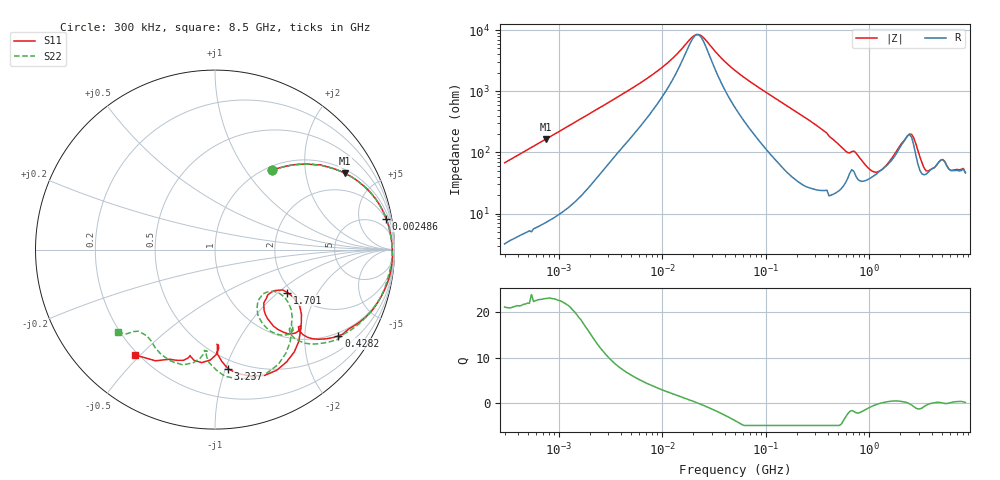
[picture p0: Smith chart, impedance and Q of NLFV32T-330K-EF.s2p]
! S-parameter Generated by TDK Corporation
! Copyright(C) 2015 TDK Corporation.
! All Rights Reserved.
! TDK P/N: NLFV32T-330K-EF (Inductors)
! Property: L=33uH at 2.52MHz
! Size(LxWxT): 3.2x2.5x2.2mm, 0.126x0.098x0.087inches
! Model Type: s2p (Touchstone File Format Version 1.0)
! Frequency: DC=Yes Start=0.3MHz Stop=8500MHz 225points Log-sweep
! Note:
! Model Generated on Jun. 23, 2015
! Hash(MD5):
! Port Assignments:
!  1 ---@@@--- 2
! Applicable Conditions:
!  Temperature = 25 degC
!  DC Bias Current = 0 A
!  Small Signal Operation
! Terms and conditions regarding TDK Simulation Models
! (1)This simulation model is being provided solely for informational purposes. Please refer to the specifications of the products in terms of detailed characteristics of such products.
! (2)In no event shall TDK Corporation of any of its subsidiaries be liable for any loss or damage arising, directly or indirectly,
!  From any information contained in this simulation model, including, but not limited to loss or damages arising from any inaccuracies, omissions or errors in connection with such information.
! (3)Any and all copyrights on this simulation model are owned by TDK Corporation.
!  Duplication or redistribution of this simulation model without prior written permission from TDK Corporation is prohibited.
! (4)This simulation model is subject to any modification or change without any prior notice.
! (5)Neither TDK Corporation nor any of its subsidiaries shall make any warranty, express or implied,
!  Including but not limited to the correctness, implied warranties of merchantability and fitness for a particular purpose with respect to this simulation models.
! (6)The use of this simulation model shall be deemed to have consented to the terms and conditions hereof.
# MHz S MA R 50
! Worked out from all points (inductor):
!   224 points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, 300 kHz to 8.5 GHz, reference 50 ohm
!   read as one part in series: L = 35.5 uH near 314.1 kHz
!   highest Q = 23 at 752.4 kHz (marker M1), where L = 34.8 uH
!   self-resonance near 21.57 MHz
!   S11 on the Smith chart (normalised r, x): 300 kHz: 1.07, +1.35; 2.486 MHz: 2, +11; 428.2 MHz: 0.90, -2.93; 1.701 GHz: 1.89, -1.16; 3.237 GHz: 0.43, -1.02; 8.5 GHz: 0.19, -0.48
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0.3  0.5464 54.1  0.8104 -33.2  0.8162 -33.4  0.5444 54.1
0.7523683  0.8388 30.5  0.5098 -57.0  0.5115 -57.3  0.8388 30.5
1.72111  0.9524 14.7  0.2561 -72.1  0.2569 -72.4  0.9532 14.6
2.486179  0.9692 10.3  0.1805 -75.1  0.1811 -75.5  0.9698 10.2
9.430415  0.9859 2.2  0.04342 -69.9  0.04346 -70.3  0.9859 2.0
21.57293  0.9887 -0.4  0.01168 -2.6  0.01167 -2.9  0.988 -0.6
51.67171  0.9887 -3.5  0.04664 72.4  0.04667 72.1  0.986 -4.0
283.1228  0.9325 -22.2  0.2965 62.3  0.2967 62.1  0.9219 -23.9
428.2171  0.8394 -35.0  0.4587 47.3  0.4591 46.9  0.8302 -37.8
618.5683  0.6525 -43.9  0.5753 24.2  0.5755 24.0  0.6271 -48.2
778.4218  0.6256 -48.8  0.5922 19.3  0.5919 19.0  0.6088 -51.7
979.5854  0.4804 -52.7  0.6611 4.1  0.6601 3.5  0.4653 -57.2
1232.735  0.3945 -43.5  0.6457 -12.3  0.6463 -12.7  0.369 -48.2
1551.304  0.4236 -32.2  0.5769 -28.6  0.5773 -29.3  0.395 -35.9
1700.7  0.4689 -30.7  0.5279 -35.1  0.5277 -35.5  0.442 -34.2
2456.696  0.7209 -52.2  0.2828 -31.4  0.2827 -32.1  0.6997 -55.7
2819.992  0.7537 -68.4  0.3506 -12.1  0.3507 -12.8  0.7459 -73.7
3237.012  0.668 -83.8  0.4868 -20.7  0.4875 -21.3  0.6719 -89.3
4465.833  0.5317 -88.0  0.4656 -55.8  0.4652 -56.3  0.5657 -95.7
5367.404  0.634 -96.7  0.3771 -58.9  0.3783 -59.8  0.667 -105.6
7072.242  0.6413 -105.9  0.3713 -79.5  0.3727 -80.2  0.6171 -130.7
8500  0.7362 -127.1  0.2815 -88.7  0.281 -87.9  0.7115 -139.7
